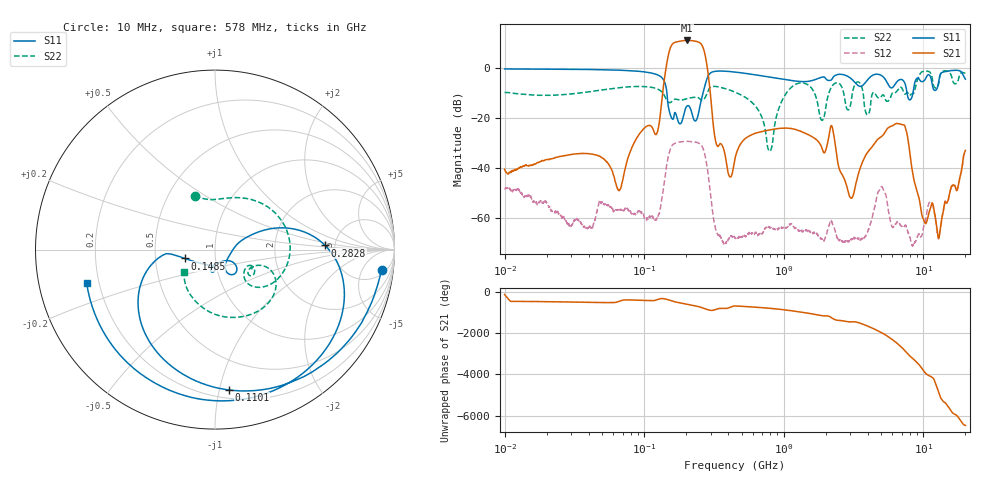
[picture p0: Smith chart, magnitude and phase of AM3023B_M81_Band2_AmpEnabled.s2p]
!Agilent Technologies,E8364B,MY43040894,A.07.50.67
!Agilent E8364B: A.07.50.67
!Date: Tuesday, October 27, 2020 10:43:07
!Correction: S11(Full 2 Port(1,2))
!S21(Full 2 Port(1,2))
!S12(Full 2 Port(1,2))
!S22(Full 2 Port(1,2))
!S2P File: Measurements: S11, S21, S12, S22:Log Frequency Sweep
# Hz S  dB  R 50
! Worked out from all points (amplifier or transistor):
!   3201 points, 10 MHz to 20 GHz, reference 50 ohm
!   highest |S21| = 10.8 dB at 202.8 MHz (marker M1)
!   |S21| within 3 dB of that: 153.9 MHz to 264.7 MHz (110.9 MHz wide, 53 % of centre)
!   unconditionally stable (mu >= 1): start of sweep to end of sweep
!   at 35.47 MHz: K = 4933.22, MAG = -25.9 dB, |S12| = -62.3 dB
!   at 447.2 MHz: K = 25040.03, MAG = -31.1 dB, |S12| = -68.0 dB
!   at 20 GHz: K = 286.58, MAG = -27.4 dB, |S12| = -33.4 dB
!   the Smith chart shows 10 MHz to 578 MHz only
!   S11 on the Smith chart (normalised r, x): 10 MHz: 7, -13; 110.1 MHz: 0.26, -1.07; 148.5 MHz: 0.71, -0.07; 282.8 MHz: 4.16, +0.31; 578 MHz: 0.15, -0.13
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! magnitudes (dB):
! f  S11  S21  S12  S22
! 10 MHz  -0.6  -40.6  -48.7  -10.0
! 35.55 MHz  -0.8  -34.3  -62.5  -10.1
! 66.08 MHz  -1.1  -49.2  -56.9  -8.1
! 110.1 MHz  -2.1  -23.2  -59.8  -7.8
! 126.1 MHz  -3.1  -24.4  -59.2  -8.7
! 148.5 MHz  -15.2  4.7  -35.6  -13.8
! 202.8 MHz  -15.4  10.8  -29.4  -12.4
! 282.8 MHz  -4.2  0.1  -40.0  -10.1
! 328.4 MHz  -1.5  -30.4  -65.1  -7.6
! 447.2 MHz  -1.8  -36.3  -68.0  -9.8
! 578 MHz  -2.6  -27.0  -65.9  -13.4
! 794.6 MHz  -3.8  -24.9  -63.9  -33.4
! 1.044 GHz  -4.9  -24.2  -64.0  -10.2
! 1.59 GHz  -5.2  -27.6  -65.3  -8.4
! 1.882 GHz  -3.8  -32.3  -68.4  -21.1
! 2.217 GHz  -4.6  -23.6  -61.7  -7.4
! 3.041 GHz  -4.5  -52.1  -68.3  -13.4
! 5.639 GHz  -7.2  -23.9  -57.8  -13.2
! 7.358 GHz  -6.2  -23.2  -63.0  -10.6
! 9.972 GHz  -5.5  -60.2  -64.4  -1.6
! 12.83 GHz  -6.1  -67.9  -68.4  -6.8
! 20 GHz  -4.7  -33.0  -33.4  -2.3
